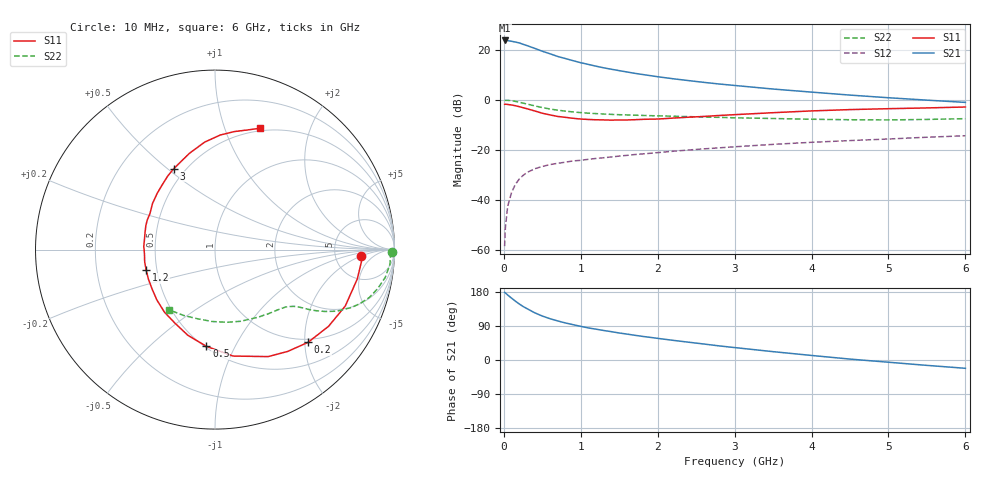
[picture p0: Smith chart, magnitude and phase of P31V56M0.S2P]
! SIEMENS Small Signal Semiconductors
! BFP181
! Si NPN RF Bipolar Junction Transistor in SOT143
! VCE = 1.5 V  IC = 6 mA
! Common Emitter S-Parameters:  March  1996
# GHz  S  MA  R  50
!  f  S11  S21  S12  S22
! GHz  MAG  ANG  MAG  ANG  MAG  ANG  MAG  ANG
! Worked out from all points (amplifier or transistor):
!   36 points, 10 MHz to 6 GHz, reference 50 ohm
!   highest |S21| = 23.7 dB at 10 MHz (marker M1)
!   |S21| within 3 dB of that: start of sweep to 387.2 MHz
!   unconditionally stable (mu >= 1): 1.338 GHz to end of sweep
!   at 250 MHz: K = 0.27, MSG = 26.2 dB, |S12| = -30.2 dB
!   at 1.4 GHz: K = 1.02, MAG = 16.6 dB, |S12| = -22.8 dB
!   at 6 GHz: K = 1.06, MAG = 5.2 dB, |S12| = -14.3 dB
!   S11 on the Smith chart (normalised r, x): 10 MHz: 9.36, -2.06; 200 MHz: 0.93, -2.07; 500 MHz: 0.51, -0.78; 1.2 GHz: 0.44, -0.12; 3 GHz: 0.43, +0.53; 6 GHz: 0.47, +1.32
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0.01  0.8152 -2.6  15.34 178.4  0.0012 83.5  0.9849 -0.9
0.02  0.8185 -4.8  15.25 177.1  0.0028 84.2  0.978 -1.8
0.05  0.8096 -11.6  15.24 171.5  0.0075 88.1  0.9784 -4.8
0.1  0.7911 -23.4  14.77 163.3  0.0141 76.0  0.9611 -9.3
0.15  0.7636 -34.0  14.25 155.3  0.0206 72.1  0.9321 -13.5
0.2  0.732 -44.9  13.71 147.9  0.0262 67.4  0.9005 -17.2
0.25  0.6969 -54.5  12.87 141.2  0.031 63.5  0.8611 -20.5
0.3  0.6656 -63.6  12.14 135.7  0.0354 59.5  0.8259 -23.0
0.4  0.6015 -80.4  10.69 124.7  0.0421 53.9  0.7588 -26.9
0.5  0.5409 -95.1  9.342 116.0  0.0468 49.2  0.7021 -29.4
0.6  0.5007 -107.6  8.317 109.0  0.0511 46.9  0.6568 -31.2
0.7  0.4664 -118.7  7.354 103.1  0.0541 45.0  0.6221 -32.5
0.9  0.4285 -139.1  6.055 93.2  0.0604 42.6  0.5738 -34.1
1.1  0.4058 -156.1  5.094 84.6  0.0651 41.6  0.5419 -35.7
1.2  0.4003 -163.3  4.694 81.3  0.0677 41.4  0.5311 -36.6
1.7  0.4018 165.7  3.391 65.3  0.0809 40.7  0.4945 -41.6
2.2  0.4327 143.5  2.639 51.9  0.0942 39.3  0.471 -48.0
3  0.5063 116.9  1.939 32.8  0.1156 35.7  0.4384 -60.8
3.5  0.5545 105.0  1.644 22.0  0.1292 32.9  0.4242 -70.3
4.5  0.6394 87.3  1.245 2.4  0.1539 26.3  0.4009 -92.3
5.5  0.6903 74.9  0.987 -14.2  0.1795 19.9  0.4066 -115.6
6  0.7201 69.8  0.89 -21.9  0.1919 16.1  0.4217 -127.3
